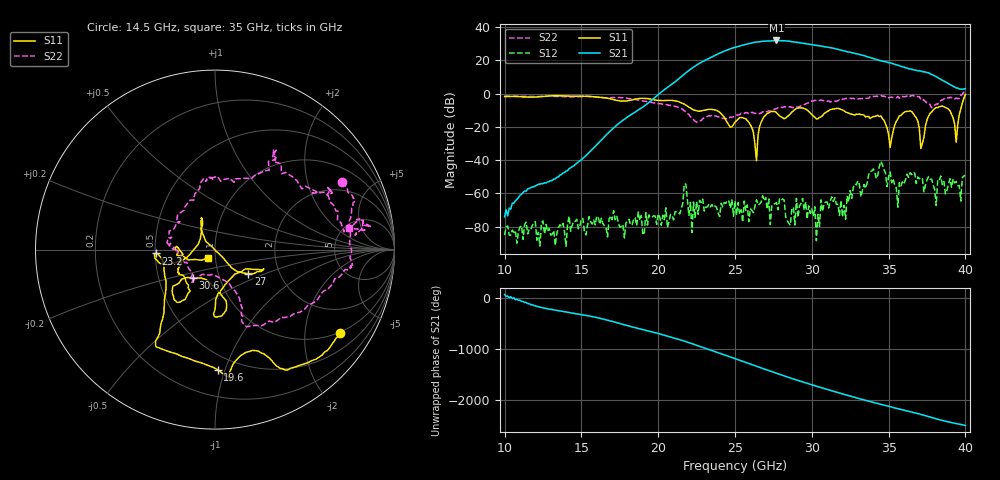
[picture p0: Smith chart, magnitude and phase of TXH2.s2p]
!Keysight Technologies,M9808A,MY58100618,A.14.70.03
!Date: Monday, February 27, 2023 13:36:51
!Correction: S11(C  2-Port  )
!S21(C  2-Port  )
!S12(C  2-Port  )
!S22(C  2-Port  )
!S2P File: Measurements: S11, S21, S12, S22:
# Hz S  RI  R 50
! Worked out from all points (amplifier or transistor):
!   301 points, 10 GHz to 40 GHz, reference 50 ohm
!   highest |S21| = 32.0 dB at 27.7 GHz (marker M1)
!   |S21| within 3 dB of that: 25.44 GHz to 30.29 GHz (4.853 GHz wide, 17.4 % of centre)
!   unconditionally stable (mu >= 1): start of sweep to 39.83 GHz
!   at 15 GHz: K = 26037.89, MAG = -29.5 dB, |S12| = -75.1 dB
!   at 25 GHz: K = 31.85, MAG = 28.1 dB, |S12| = -64.5 dB
!   at 40 GHz: K = -7.59, MSG = 26.1 dB, |S12| = -49.1 dB
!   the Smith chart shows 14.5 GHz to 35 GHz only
!   S11 on the Smith chart (normalised r, x): 14.5 GHz: 0.98, -3.04; 19.6 GHz: 0.39, -0.94; 23.2 GHz: 0.50, -0.02; 27 GHz: 1.39, -0.39; 30.6 GHz: 0.75, -0.24; 35 GHz: 0.92, -0.08
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1e10  0.7353 0.3667  7.39e-05 0.000185  -5.57e-05 6.5e-06  0.028 0.8382
1.45e10  0.6985 -0.4622  0.00319 0.00591  -0.000123 7.49e-05  0.7078 0.3765
1.5e10  0.6388 -0.5462  0.00848 0.00593  0.000176 -1.26e-05  0.7657 0.2994
1.96e10  0.0147 -0.6688  0.341 0.551  -0.000121 0.000152  0.3844 -0.3792
2e10  -0.1099 -0.6215  0.8391 0.4223  -9.46e-05 0.000225  0.3004 -0.3979
2.19e10  -0.2827 -0.3117  -3.6 -2.876  0.000622 -5.11e-05  0.1116 -0.2299
2.32e10  -0.3305 -0.0216  1.177 10.89  0.000218 0.000325  -0.1184 -0.1708
2.42e10  -0.2113 -0.0694  17.09 -6.047  1.57e-05 -0.000393  -0.1301 -0.1263
2.5e10  -0.0755 0.1179  -6.386 -23.83  -0.000475 0.000361  -0.2103 -0.00573
2.59e10  -0.0764 0.1138  -30.17 11.01  -0.000137 4.15e-05  -0.2412 0.0688
2.65e10  0.0403 -0.04  -3.612 36.13  0.000177 -0.000409  -0.2162 0.1419
2.7e10  0.1866 -0.1339  28.12 25.82  0.000339 -0.000672  -0.1715 0.2208
2.77e10  0.2467 -0.1112  34.24 -20.48  -0.000531 1.21e-05  -0.0844 0.3421
2.83e10  0.0809 -0.1673  -1.734 -38.76  0.000191 -4.74e-05  -0.0167 0.3987
2.9e10  -0.0079 -0.3572  -33.42 -10.97  7.62e-05 0.000708  0.0828 0.3975
3e10  0.024 -0.2367  -6.888 29.09  0.000311 0.000147  0.3374 0.5015
3.06e10  -0.1241 -0.1568  17.7 20.43  0.000504 -0.000394  0.3244 0.5574
3.12e10  -0.2388 -0.2269  24.09 -1.976  -3.32e-05 -0.000575  0.3697 0.4228
3.2e10  -0.166 -0.2778  5.226 -19.02  -0.000186 6.99e-05  0.6077 0.3197
3.32e10  -0.204 -0.112  -14.73 -1.212  0.000758 0.000232  0.6738 0.216
3.5e10  -0.0378 -0.0448  6.271 5.976  8.81e-05 -0.00323  0.7473 0.1181
4e10  0.4694 -0.8284  1.236 0.6876  -0.00298 0.00183  1.154 -0.6896
